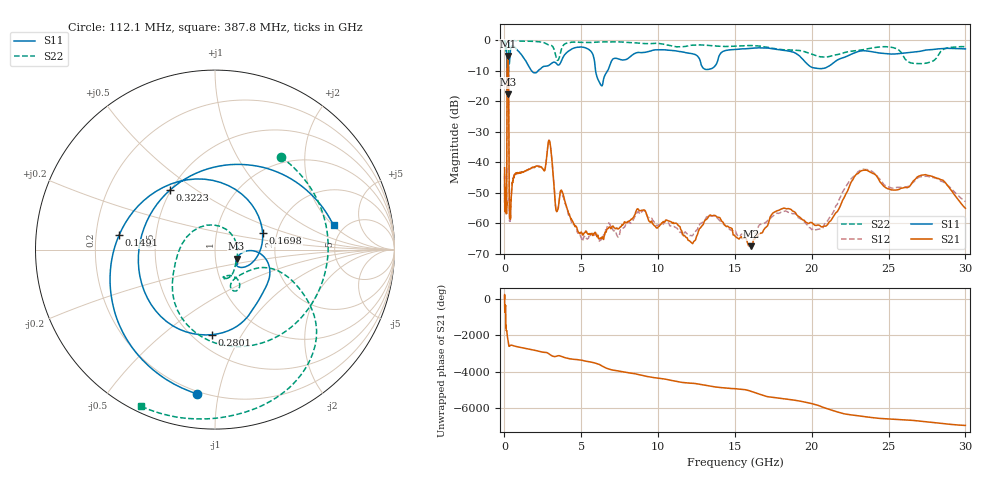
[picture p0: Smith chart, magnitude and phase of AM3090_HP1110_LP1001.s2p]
! Date/Time: Thu, Feb 28, 2019 2:09 PM
! Network Analyzer: Agilent Technologies E8364B Rev: A.07.50.67
! Sweep from 0.010 to 30.000 GHz, 1601 Points, Sweep Type: LOG
! Power Supply: 5.023 V, 0.002 A
# Hz S DB R 50
!freq MagS11 AngS11 MagS21 AngS21 MagS12 AngS12 MagS22 AngS22
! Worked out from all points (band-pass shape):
!   1601 points, 10 MHz to 30 GHz, reference 50 ohm
!   highest |S21| = -5.15 dB at 212.7 MHz (marker M1); lowest = -67.4 dB at 16.05 GHz (marker M2)
!   |S21| within 3 dB of the highest: 175.1 MHz to 256.3 MHz (81.27 MHz wide, 37.7 % of centre)
!   lowest |S11| = -17.7 dB at 213.8 MHz (marker M3), VSWR 1.30, Z = 63.3 - j6.39 ohm
!   |S11| at or under -10 dB: 166.3 MHz to 238.4 MHz (72.06 MHz wide, 35.6 % of centre); 1.763 GHz to 2.2 GHz (437 MHz wide, 22.1 % of centre); 5.93 GHz to 6.719 GHz (789.4 MHz wide, 12.5 % of centre)
!   |S22| runs from -18.1 to -0.1 dB; largest |S21 - S12| = 0.013
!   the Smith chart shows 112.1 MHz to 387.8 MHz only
!   S11 on the Smith chart (normalised r, x): 112.1 MHz: 0.19, -0.87; 149.1 MHz: 0.30, +0.07; 169.8 MHz: 1.68, +0.33; 280.1 MHz: 0.61, -0.75; 322.3 MHz: 0.49, +0.40; 387.8 MHz: 4.10, +2.02
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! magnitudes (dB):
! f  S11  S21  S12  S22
! 10 MHz  -0.3  -41.8  -48.9  -0.7
! 22.38 MHz  -0.9  -56.0  -51.6  -1.1
! 38.04 MHz  -0.3  -50.9  -50.2  -1.3
! 112.1 MHz  -1.8  -53.8  -53.6  -4.0
! 144.7 MHz  -4.5  -49.9  -48.7  -4.8
! 149.1 MHz  -5.3  -41.8  -41.9  -5.5
! 169.8 MHz  -11.0  -10.6  -10.6  -18.1
! 212.7 MHz  -17.7  -5.1  -5.1  -15.9
! 213.8 MHz  -17.7  -5.2  -5.1  -15.9
! 258.6 MHz  -8.6  -8.6  -8.6  -13.9
! 280.1 MHz  -6.5  -24.1  -24.1  -5.3
! 322.3 MHz  -7.6  -55.4  -58.3  -0.7
! 387.8 MHz  -3.4  -58.6  -57.8  -0.3
! 550.5 MHz  -2.0  -46.1  -45.3  -0.2
! 2.084 GHz  -10.6  -41.2  -41.2  -0.5
! 2.913 GHz  -8.2  -32.8  -32.8  -1.6
! 3.402 GHz  -7.8  -56.2  -56.1  -6.3
! 7.926 GHz  -6.3  -59.7  -60.1  -0.7
! 16.05 GHz  -2.7  -67.4  -63.5  -1.8
! 20.51 GHz  -9.3  -60.6  -61.8  -5.4
! 23.36 GHz  -3.5  -42.6  -42.2  -3.1
! 30 GHz  -2.9  -55.0  -52.9  -2.2
